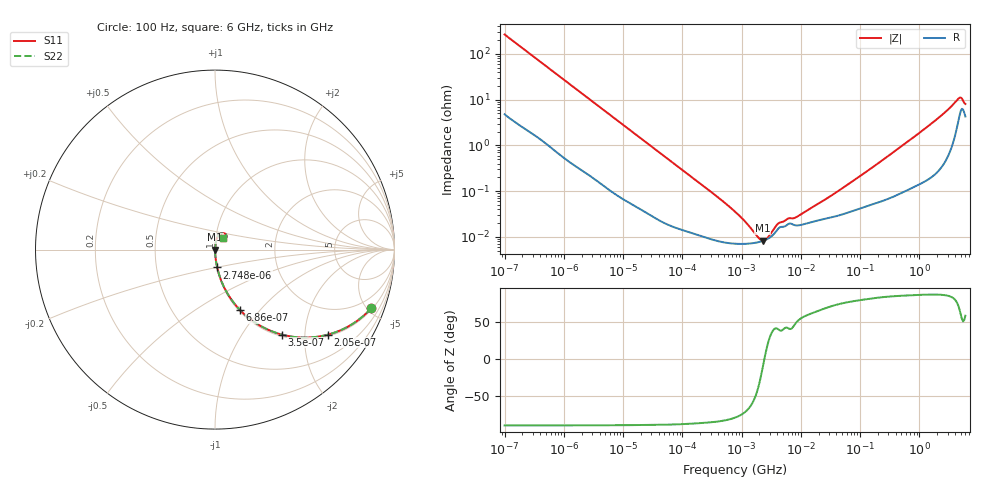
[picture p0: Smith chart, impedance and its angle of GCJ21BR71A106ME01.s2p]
!Murata Part Number: GCJ21BR71A106ME01
!These Parameters are Measured in Series Mode Connection
!Data Generated on Mar 13, 2026
!  o--ll--o
!Port1  Port2
!  o------o
!Operation Temp=25[degC], DC Bias Voltage=0[V]
!Freq. Start=100[Hz] Stop=6[GHz] 401[Steps]
# Hz S RI R 50
!Freq.(Hz) S11(Real) S11(Imag) S21(Real) S21(Imag) S12(Real) S12(Imag) S22(Real) S22(Imag)
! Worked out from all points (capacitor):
!   401 points, 100 Hz to 6 GHz, reference 50 ohm
!   read as one part in series: C = 5.98 uF near 109 Hz
!   lowest |Z| = 8.33 mohm at 2.269 MHz (marker M1)
!   series resonance near 2.427 MHz, so ESL is about 720 pH
!   S11 on the Smith chart (normalised r, x): 100 Hz: 1.10, -5.31; 205 Hz: 1.05, -2.61; 350 Hz: 1.03, -1.54; 686 Hz: 1.02, -0.79; 2.748 kHz: 1.00, -0.20; 6 GHz: 1.09, +0.14
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100  0.8712 -0.3261  0.1288 0.3261  0.1288 0.3261  0.8712 -0.3261
205  0.6281 -0.474  0.3719 0.474  0.3719 0.474  0.6281 -0.474
350  0.3738 -0.4739  0.6262 0.4739  0.6262 0.4739  0.3738 -0.4739
686  0.1406 -0.3379  0.8594 0.3379  0.8594 0.3379  0.1406 -0.3379
2008  0.0211 -0.1337  0.9789 0.1337  0.9789 0.1337  0.0211 -0.1337
2748  0.0121 -0.0991  0.9879 0.0991  0.9879 0.0991  0.0121 -0.0991
8047  0.002 -0.0347  0.998 0.0347  0.998 0.0347  0.002 -0.0347
40335  0.000282 -0.00711  0.9997 0.00711  0.9997 0.00711  0.000282 -0.00711
774597  7.11e-05 -0.00035  0.9999 0.00035  0.9999 0.00035  7.11e-05 -0.00035
1813585  7.55e-05 -7.4e-05  0.9999 7.4e-05  0.9999 7.4e-05  7.55e-05 -7.4e-05
2268635  8.15e-05 -1.7e-05  0.9999 1.7e-05  0.9999 1.7e-05  8.15e-05 -1.7e-05
2837864  9.26e-05 3.97e-05  0.9999 -3.97e-05  0.9999 -3.97e-05  9.26e-05 3.97e-05
4246196  0.000156 0.000127  0.9998 -0.000127  0.9998 -0.000127  0.000156 0.000127
6075234  0.000189 0.000167  0.9998 -0.000167  0.9998 -0.000167  0.000189 0.000167
8311524  0.000179 0.000201  0.9998 -0.000201  0.9998 -0.000201  0.000179 0.000201
1.555665e7  0.000213 0.000389  0.9998 -0.000389  0.9998 -0.000389  0.000213 0.000389
4.764863e7  0.000305 0.00106  0.9997 -0.00106  0.9997 -0.00106  0.000305 0.00106
3.124326e8  0.000732 0.00608  0.9993 -0.00608  0.9993 -0.00608  0.000732 0.00608
1.791126e9  0.00337 0.0334  0.9966 -0.0334  0.9966 -0.0334  0.00337 0.0334
4.586474e9  0.0427 0.0921  0.9573 -0.0921  0.9573 -0.0921  0.0427 0.0921
5.016141e9  0.0614 0.0849  0.9386 -0.0849  0.9386 -0.0849  0.0614 0.0849
6e9  0.0452 0.0624  0.9548 -0.0624  0.9548 -0.0624  0.0452 0.0624
